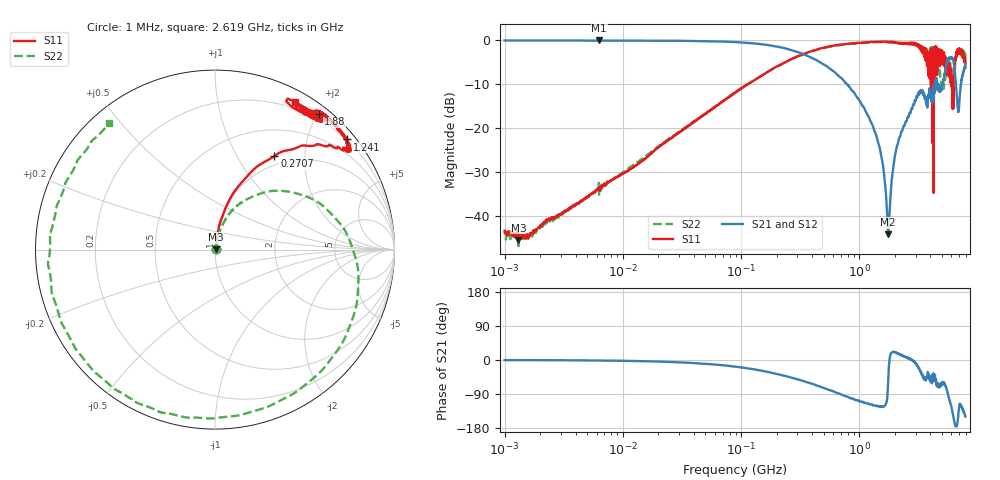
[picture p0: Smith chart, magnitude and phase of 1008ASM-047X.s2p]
!s-Parameter Generated by FASTRON Sdn. Bhd.
!FASTRON P/N : 1008ASM-047X
!Keysight Technologies: E5071C_MY46733604_B.14.02
!Date: Tue Nov 21 11:27:24 2023
!Version  :Rev00  Wed Nov 22 15:48:28 2023
!Data & Calibration Information:
!Freq  S11:SOLT2(ON)  S21:SOLT2(ON)  S12:SOLT2(ON)  S22:SOLT2(ON)
!PortZ  Port1:50+j0  Port2:50+j0
!When reading reference impedance value at option line is always used.
! Remarks : This data is being provided solely for informational purposes.
# Hz S dB R 50
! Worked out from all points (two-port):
!   1599 points, 1 MHz to 7.923 GHz, reference 50 ohm
!   highest |S21| = -0.03 dB at 6.301 MHz (marker M1); lowest = -44.1 dB at 1.763 GHz (marker M2)
!   |S21| within 3 dB of the highest: start of sweep to 330.2 MHz
!   lowest |S11| = -45.4 dB at 1.31 MHz (marker M3), VSWR 1.01, Z = 50.5 + j0.183 ohm
!   |S11| at or under -10 dB: start of sweep to 113.7 MHz; 4.043327 GHz to 4.060218 GHz (16.89 MHz wide, 0.417 % of centre); 6.117 GHz to 6.296 GHz (179.6 MHz wide, 2.89 % of centre)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
!   |S22| runs from -46.8 to -0.4 dB; largest |S21 - S12| = 0.011
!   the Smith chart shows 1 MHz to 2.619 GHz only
!   S11 on the Smith chart (normalised r, x): 1 MHz: 1.01, +0.00; 270.7 MHz: 0.86, +1.45; 1.241 GHz: 0.18, +2.75; 1.88 GHz: 0.13, +2.02; 2.619 GHz: 0.13, +1.67
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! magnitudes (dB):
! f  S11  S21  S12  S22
! 1 MHz  -43.3  0.0  -0.1  -43.5
! 1.31 MHz  -45.4  -0.1  0.0  -46.8
! 4.479 MHz  -36.4  -0.1  -0.1  -36.6
! 6.301 MHz  -33.7  0.0  -0.1  -35.4
! 19.95 MHz  -24.3  -0.1  -0.1  -24.2
! 89.01 MHz  -11.9  -0.4  -0.4  -11.9
! 270.7 MHz  -4.2  -2.3  -2.3  -4.2
! 398.5 MHz  -2.4  -4.0  -4.0  -2.5
! 1.241 GHz  -0.4  -18.3  -18.3  -0.5
! 1.543 GHz  -0.3  -26.5  -26.5  -0.4
! 1.763 GHz  -0.3  -44.1  -44.1  -0.5
! 1.784 GHz  -0.4  -42.4  -42.4  -0.5
! 1.88 GHz  -0.5  -32.1  -32.2  -0.6
! 2.114 GHz  -0.5  -23.7  -23.7  -0.7
! 2.619 GHz  -0.6  -17.5  -17.5  -0.7
! 3.224 GHz  -1.1  -12.0  -12.0  -1.3
! 4.325 GHz  -1.7  -11.3  -11.3  -2.1
! 5.08 GHz  -5.5  -9.7  -9.7  -11.1
! 5.668 GHz  -7.6  -4.1  -4.1  -5.2
! 6.034 GHz  -9.6  -3.9  -3.9  -7.9
! 6.92 GHz  -2.1  -16.3  -16.2  -2.6
! 7.923 GHz  -6.2  -5.4  -5.4  -4.2
